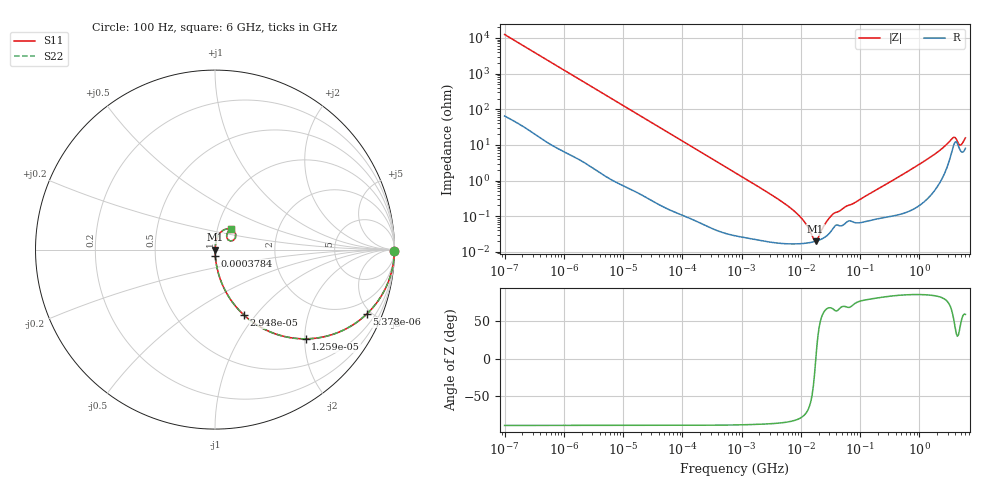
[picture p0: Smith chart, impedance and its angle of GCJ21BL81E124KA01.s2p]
!Murata Part Number: GCJ21BL81E124KA01
!These Parameters are Measured in Series Mode Connection
!Data Generated on Mar 13, 2026
!  o--ll--o
!Port1  Port2
!  o------o
!Operation Temp=25[degC], DC Bias Voltage=0[V]
!Freq. Start=100[Hz] Stop=6[GHz] 401[Steps]
# Hz S RI R 50
!Freq.(Hz) S11(Real) S11(Imag) S21(Real) S21(Imag) S12(Real) S12(Imag) S22(Real) S22(Imag)
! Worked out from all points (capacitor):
!   401 points, 100 Hz to 6 GHz, reference 50 ohm
!   read as one part in series: C = 127 nF near 109 Hz
!   lowest |Z| = 19.8 mohm at 17.79 MHz (marker M1)
!   series resonance near 17.92 MHz, so ESL is about 620 pH
!   S11 on the Smith chart (normalised r, x): 100 Hz: open; 5.378 kHz: 1.02, -4.72; 12.59 kHz: 1.01, -2.02; 29.48 kHz: 1.01, -0.87; 378.4 kHz: 1.00, -0.07; 6 GHz: 1.16, +0.27
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100  0.9999 -0.00798  0.000105 0.00798  0.000105 0.00798  0.9999 -0.00798
2008  0.9746 -0.1546  0.0254 0.1546  0.0254 0.1546  0.9746 -0.1546
5378  0.8465 -0.3579  0.1535 0.3579  0.1535 0.3579  0.8465 -0.3579
12592  0.5052 -0.497  0.4948 0.497  0.4948 0.497  0.5052 -0.497
29482  0.1596 -0.363  0.8404 0.363  0.8404 0.363  0.1596 -0.363
40335  0.0928 -0.2869  0.9072 0.2869  0.9072 0.2869  0.0928 -0.2869
108014  0.0149 -0.1169  0.9851 0.1169  0.9851 0.1169  0.0149 -0.1169
378399  0.00156 -0.034  0.9984 0.034  0.9984 0.034  0.00156 -0.034
774597  0.00056 -0.0167  0.9994 0.0167  0.9994 0.0167  0.00056 -0.0167
7266822  0.000169 -0.00151  0.9998 0.00151  0.9998 0.00151  0.000169 -0.00151
1.137099e7  0.000173 -0.000692  0.9998 0.000692  0.9998 0.000692  0.000173 -0.000692
1.555665e7  0.000187 -0.000209  0.9998 0.000209  0.9998 0.000209  0.000187 -0.000209
1.779312e7  0.000197 -1.06e-05  0.9998 1.06e-05  0.9998 1.06e-05  0.000197 -1.06e-05
1.946e7  0.000207 0.000122  0.9998 -0.000122  0.9998 -0.000122  0.000207 0.000122
2.662322e7  0.00027 0.000609  0.9997 -0.000609  0.9997 -0.000609  0.00027 0.000609
3.482834e7  0.00045 0.00105  0.9995 -0.00105  0.9995 -0.00105  0.00045 0.00105
3.124326e8  0.00104 0.00881  0.999 -0.00881  0.999 -0.00881  0.00104 0.00881
1.565993e9  0.00595 0.0456  0.994 -0.0456  0.994 -0.0456  0.00595 0.0456
3.505958e9  0.0714 0.1156  0.9286 -0.1156  0.9286 -0.1156  0.0714 0.1156
4.009986e9  0.1151 0.0863  0.8849 -0.0863  0.8849 -0.0863  0.1151 0.0863
5.016141e9  0.0668 0.0638  0.9332 -0.0638  0.9332 -0.0638  0.0668 0.0638
6e9  0.0885 0.1141  0.9115 -0.1141  0.9115 -0.1141  0.0885 0.1141
